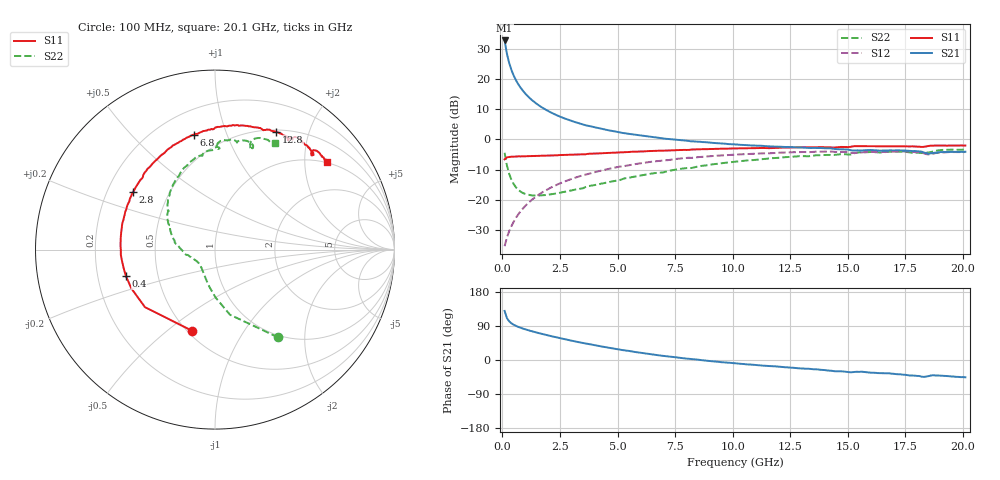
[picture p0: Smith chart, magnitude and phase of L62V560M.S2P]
!  Infineon Technologies AG
! BFR380L3 , PF131585-7, No.6, Th 09.10.01, soldered on pcb-board, measured with PP GSG850
!  Vce=2.5 V,  Ic=60.0 mA
! Common Emitter S-Parameters:  15. November 2001
#  GHz  S  MA  R  50
! f  S11  S21  S12  S22
! GHz  Mag  Ang  Mag  Ang  Mag  Ang  Mag  Ang
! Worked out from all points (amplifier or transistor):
!   201 points, 100 MHz to 20.1 GHz, reference 50 ohm
!   highest |S21| = 32.7 dB at 100 MHz (marker M1)
!   |S21| within 3 dB of that: start of sweep to 168.5 MHz
!   unconditionally stable (mu >= 1): 791.2 MHz to 4.26 GHz; 18.35 GHz to 18.53 GHz
!   at 3.4 GHz: K = 1.02, MAG = 7.8 dB, |S12| = -12.1 dB
!   at 10.1 GHz: K = 0.96, MSG = 1.7 dB, |S12| = -5.0 dB
!   at 20.1 GHz: K = 0.99, MSG = 0.0 dB, |S12| = -4.2 dB
!   S11 on the Smith chart (normalised r, x): 100 MHz: 0.53, -0.61; 400 MHz: 0.32, -0.13; 2.8 GHz: 0.31, +0.29; 6.8 GHz: 0.35, +0.77; 12.8 GHz: 0.52, +1.52; 20.1 GHz: 0.98, +2.56
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0.1  0.4695 -106.1  43.07 129.5  0.01729 58.1  0.602 -54.3
0.2  0.5051 -140.6  26.02 110.5  0.02402 57.9  0.3723 -77.0
0.3  0.5136 -155.1  18.18 101.9  0.03076 61.8  0.2685 -89.1
0.4  0.5179 -163.5  13.9 96.6  0.03726 64.3  0.2137 -97.8
0.5  0.5195 -169.0  11.2 92.8  0.04412 66.7  0.1813 -104.7
0.6  0.5222 -173.3  9.38 89.8  0.05136 68.0  0.1607 -110.3
0.7  0.5255 -177.0  8.086 87.2  0.05836 69.0  0.1468 -115.5
0.8  0.5245 -179.9  7.092 84.9  0.06572 69.8  0.1371 -119.9
0.9  0.527 177.4  6.319 82.8  0.07283 70.0  0.1301 -123.6
1.1  0.5292 172.9  5.202 79.0  0.08745 70.3  0.123 -130.4
1.4  0.5329 167.0  4.115 73.9  0.1092 69.6  0.1184 -138.3
1.8  0.5384 160.1  3.235 67.7  0.1384 67.9  0.1196 -146.3
2.3  0.5477 152.3  2.574 60.4  0.1739 65.1  0.1275 -154.8
2.8  0.5584 145.2  2.154 53.7  0.2087 61.9  0.1389 -161.6
3.5  0.5679 135.8  1.766 44.8  0.2564 57.0  0.156 -169.1
5.1  0.6086 117.4  1.307 27.2  0.3559 45.2  0.2134 171.9
6.8  0.6515 100.5  1.059 12.2  0.4436 33.1  0.2829 152.5
10.1  0.7095 76.4  0.8282 -8.7  0.5604 11.1  0.4286 123.3
12.8  0.7411 62.6  0.741 -21.5  0.6175 -5.7  0.5269 101.4
13.5  0.7417 59.5  0.7254 -24.3  0.6227 -9.5  0.5394 97.0
16.8  0.7735 47.3  0.6608 -35.2  0.6274 -25.4  0.6249 76.5
20.1  0.7912 38.1  0.627 -45.6  0.62 -38.9  0.6789 60.8
